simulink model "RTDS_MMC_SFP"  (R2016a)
settings: Solver=FixedStepAuto  StartTime=0.0  StopTime=0.4  RelTol=1e-3
PreLoadFcn:
  | % --- DO NOT REMOVE THIS CODE (2024.3.b1) ---
  |     % create Simulink variants
  |     if not(exist('variant_simulation', 'var'))
  |         variant_simulation = Simulink.Variant('SIMULINK_MODE==0');
  |     end
  |     if not(exist('variant_generation', 'var'))
  |         variant_generation = Simulink.Variant('SIMULINK_MODE==1');
  |     end
  | 
  |     % check SDK version
  |     required_lib_version = 3900.3;
  |     required_lib_ver_str = '2024.3';
  |     lib_path = [getenv('IX_SIMULINK_ACG_BB_3') '\simulink\blocks\BoomBox.slx'];
  |     if exist(lib_path, 'file')
  |         lib_version = str2double(Simulink.MDLInfo(lib_path).ModelVersion); % fullpath to avoid getting shadowing files
  |         if lib_version < required_lib_version || isnan(lib_version)
  |             error(['The model ''' bdroot ''' has been saved with a more recent version of ACG SDK (' required_lib_ver_str ') and might not work as expected. <a href="matlab:private_end_string = ''--- PLACE YOUR CODE BELOW THIS LINE ---'';private_fcn = get_param(bdroot, ''PreLoadFcn'');private_end_index = strfind(private_fcn, private_end_string);set_param(bdroot, ''PreLoadFcn'', strtrim(private_fcn(private_end_index(end)+length(private_end_string):end)));private_fcn = get_param(bdroot, ''PostLoadFcn'');private_end_index = strfind(private_fcn, private_end_string);set_param(bdroot, ''PostLoadFcn'', strtrim(private_fcn(private_end_index(end)+length(private_end_string):end)));private_fcn = get_param(bdroot, ''InitFcn'');private_end_index = strfind(private_fcn, private_end_string);set_param(bdroot, ''InitFcn'', strtrim(private_fcn(private_end_index(end)+length(private_end_string):end)));clear private_end_string private_fcn private_end_index;open(bdroot);">Click here</a> to continue anyway, or download the latest version of the SDK at <a href="www.imperix.com/downloads">www.imperix.ch/downloads</a>.']);
  |         end
  |     elseif exist(getenv('IX_SIMULINK_ACG_BB_3'), 'dir')
  |         error(['Library file for imperix ACG SDK not found in path ''' lib_path '''. Please try to re-install ACG SDK (<a href="www.imperix.com/downloads">www.imperix.ch/downloads</a>).']);
  |     else
  |         error('ACG SDK is not installed on this computer and the model will not work as expected. Please download ACG SDK at <a href="www.imperix.com/downloads">www.imperix.ch/downloads</a>, install it, and reopen the model.');
  |     end
  |     clear required_lib_version required_lib_ver_str lib_path lib_version;
  | 
  |     ix_acg_path = getenv('IX_SIMULINK_ACG_BB_3');
  |     addpath(fullfile(ix_acg_path, 'simulink\target'));
  |     addpath(fullfile(ix_acg_path, 'simulink\blocks'));
  |     addpath(fullfile(ix_acg_path, 'simulink\functions'));
  |     sl_refresh_customizations;
  |     clear ix_acg_path;
  | 
  |     % The SIMULINK_MODE variable is created in the base
  |     % workspace in the PostLoadFcn from the block whose id is kb0101
  |     % All opened models share a common variant configuration.
  | 
  |     Model_PreLoadFcn(bdroot);
  | % --- PLACE YOUR CODE BELOW THIS LINE ---
PostLoadFcn:
  | % --- DO NOT REMOVE THIS CODE (2024.3.b1) ---
  |     % change the execution mode of simulink depending on the radio button:
  |     if(strcmp('Automated Code Generation',get_param(Find_imperix_blocks(bdroot,'Configuration'),'SLMODE')))
  |         assignin('base', 'SIMULINK_MODE', 1);
  |     else
  |         assignin('base', 'SIMULINK_MODE', 0);
  |     end
  | 
  |     Model_PostLoadFcn(bdroot);
  | % --- PLACE YOUR CODE BELOW THIS LINE ---
InitFcn:
  | % --- DO NOT REMOVE THIS CODE (2024.3.b1) ---
  |     % check SDK version
  |     required_lib_version = 3900.3;
  |     required_lib_ver_str = '2024.3';
  |     lib_path = [getenv('IX_SIMULINK_ACG_BB_3') '\simulink\blocks\BoomBox.slx'];
  |     if exist(lib_path, 'file')
  |         lib_version = str2double(Simulink.MDLInfo(lib_path).ModelVersion); % fullpath to avoid getting shadowing files
  |         if lib_version < required_lib_version || isnan(lib_version)
  |             error(['The model ''' bdroot ''' has been saved with a more recent version of ACG SDK (' required_lib_ver_str ') and might not work as expected. <a href="matlab:private_end_string = ''--- PLACE YOUR CODE BELOW THIS LINE ---'';private_fcn = get_param(bdroot, ''PreLoadFcn'');private_end_index = strfind(private_fcn, private_end_string);set_param(bdroot, ''PreLoadFcn'', strtrim(private_fcn(private_end_index(end)+length(private_end_string):end)));private_fcn = get_param(bdroot, ''PostLoadFcn'');private_end_index = strfind(private_fcn, private_end_string);set_param(bdroot, ''PostLoadFcn'', strtrim(private_fcn(private_end_index(end)+length(private_end_string):end)));private_fcn = get_param(bdroot, ''InitFcn'');private_end_index = strfind(private_fcn, private_end_string);set_param(bdroot, ''InitFcn'', strtrim(private_fcn(private_end_index(end)+length(private_end_string):end)));clear private_end_string private_fcn private_end_index;open(bdroot);">Click here</a> to continue anyway, or download the latest version of the SDK at <a href="www.imperix.com/downloads">www.imperix.ch/downloads</a>.']);
  |         end
  |     elseif exist(getenv('IX_SIMULINK_ACG_BB_3'), 'dir')
  |         error(['Library file for imperix ACG SDK not found in path ''' lib_path '''. Please try to re-install ACG SDK (<a href="www.imperix.com/downloads">www.imperix.ch/downloads</a>).']);
  |     else
  |         error('ACG SDK is not installed on this computer and the model will not work as expected. Please download ACG SDK at <a href="www.imperix.com/downloads">www.imperix.ch/downloads</a>, install it, and reopen the model.');
  |     end
  |     clear required_lib_version required_lib_ver_str lib_path lib_version;
  | 
  |     Model_InitFcn(bdroot);
  | % --- PLACE YOUR CODE BELOW THIS LINE ---
model workspace (MAT data in the model file):
  CTRLPERIOD = 0.0002
  TSAMPLE = 2e-06
  global_CLK_number = 0
  global_INT_number = 1
  global_SVM_instance_id = 0
  global_can_baud_rate = '1000000'
  global_comp_time = 0.2
  global_cycle_delay = 8e-05
  global_ip_addresses : cell (value not decoded)
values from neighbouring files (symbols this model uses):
  Ki_Vleg = 1/Ti    (= 2.95256991686)    [RTDS_MMC_SFP_init.m]
  Kp_Vleg = Tn/Ti    (= 0.14880952381)    [RTDS_MMC_SFP_init.m]
  N = 4    [RTDS_MMC_SFP_init.m]
  scale_factor = 0.5^16    (= 1.52587890625e-05)    [RTDS_MMC_SFP_init.m]
  Tsw = 1/fsw    (= 0.0008)    [RTDS_MMC_SFP_init.m]
  Vsm_max = 250    [RTDS_MMC_SFP_init.m]
undefined symbols (not defined in the file or in its folder): B, Board, Box, channel, DT, lane, Micro, ns, PRO, RCP, TPI, Vf
libraries: BoomBox x183, simulink x55
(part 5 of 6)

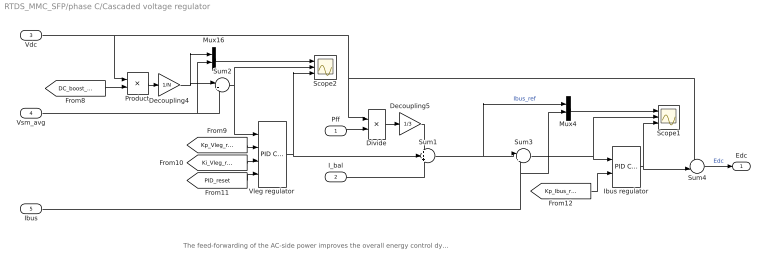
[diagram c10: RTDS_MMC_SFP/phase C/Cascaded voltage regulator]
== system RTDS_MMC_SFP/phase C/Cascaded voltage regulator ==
  note: The feed-forwarding of the AC-side power improves the overall energy control dynamics.
  Pff : Inport
  I_bal : Inport  Port=2
  Vdc : Inport  Port=3
  Vsm_avg : Inport  Port=4
  Ibus : Inport  Port=5
  Decoupling4 : Gain  Gain=1/N
  Decoupling5 : Gain  Gain=1/3
  Divide : Product  Inputs=/*
  Ibus regulator : simulink/Continuous/PID Controller  Controller=P  TimeDomain=Discrete-time  SampleTime=-1  IntegratorMethod=Forward Euler  FilterMethod=Forward Euler  Form=Parallel  UseFilter=on  ControllerParametersSource=external  P=8  I=0.5  D=0  N=100  InitialConditionSource=internal  InitialConditionForIntegrator=0  InitialConditionForFilter=0  ExternalReset=none  LimitOutput=off  UpperSaturationLimit=inf  LowerSaturationLimit=-inf  LinearizeAsGain=off  AntiWindupMode=none  Kb=1  TrackingMode=off  Kt=1  PParamMin=[]  PParamMax=[]  IParamMin=[]  IParamMax=[]  DParamMin=[]  DParamMax=[]  NParamMin=[]  NParamMax=[]  KbParamMin=[]  KbParamMax=[]  KtParamMin=[]  KtParamMax=[]  POutMin=[]  POutMax=[]  IOutMin=[]  IOutMax=[]  DOutMin=[]  DOutMax=[]  NOutMin=[]  NOutMax=[]  KbOutMin=[]  KbOutMax=[]  KtOutMin=[]  KtOutMax=[]  IntegratorOutMin=[]  IntegratorOutMax=[]  FilterOutMin=[]  FilterOutMax=[]  SumOutMin=[]  SumOutMax=[]  SumI1OutMin=[]  SumI1OutMax=[]  SumI2OutMin=[]  SumI2OutMax=[]  SumI3OutMin=[]  SumI3OutMax=[]  SumDOutMin=[]  SumDOutMax=[]  SaturationOutMin=[]  SaturationOutMax=[]  IntegratorContinuousStateAttributes=''  IntegratorStateMustResolveToSignalObject=off  IntegratorRTWStateStorageClass=Auto  FilterContinuousStateAttributes=''  FilterStateMustResolveToSignalObject=off  FilterRTWStateStorageClass=Auto  DifferentiatorICPrevScaledInput=0  DifferentiatorOutMin=[]  DifferentiatorOutMax=[]
  Mux16 : Mux  Inputs=2
  Mux4 : Mux  Inputs=2
  Product : Product
  Scope1 : Scope  NumInputPorts=3
  Scope2 : Scope  NumInputPorts=3
  Sum1 : Sum  Inputs=+++
  Sum2 : Sum  Inputs=|+-
  Sum3 : Sum  Inputs=|+-
  Sum4 : Sum  Inputs=+-|
  Vleg regulator : simulink/Continuous/PID Controller  Controller=PI  TimeDomain=Discrete-time  SampleTime=-1  IntegratorMethod=Forward Euler  FilterMethod=Forward Euler  Form=Parallel  UseFilter=on  ControllerParametersSource=external  P=8  I=0.5  D=0  N=100  InitialConditionSource=internal  InitialConditionForIntegrator=0  InitialConditionForFilter=0  ExternalReset=level  LimitOutput=on  UpperSaturationLimit=10  LowerSaturationLimit=-10  LinearizeAsGain=off  AntiWindupMode=back-calculation  Kb=Ki_Vleg/Kp_Vleg  TrackingMode=off  Kt=1  PParamMin=[]  PParamMax=[]  IParamMin=[]  IParamMax=[]  DParamMin=[]  DParamMax=[]  NParamMin=[]  NParamMax=[]  KbParamMin=[]  KbParamMax=[]  KtParamMin=[]  KtParamMax=[]  POutMin=[]  POutMax=[]  IOutMin=[]  IOutMax=[]  DOutMin=[]  DOutMax=[]  NOutMin=[]  NOutMax=[]  KbOutMin=[]  KbOutMax=[]  KtOutMin=[]  KtOutMax=[]  IntegratorOutMin=[]  IntegratorOutMax=[]  FilterOutMin=[]  FilterOutMax=[]  SumOutMin=[]  SumOutMax=[]  SumI1OutMin=[]  SumI1OutMax=[]  SumI2OutMin=[]  SumI2OutMax=[]  SumI3OutMin=[]  SumI3OutMax=[]  SumDOutMin=[]  SumDOutMax=[]  SaturationOutMin=[]  SaturationOutMax=[]  IntegratorContinuousStateAttributes=''  IntegratorStateMustResolveToSignalObject=off  IntegratorRTWStateStorageClass=Auto  FilterContinuousStateAttributes=''  FilterStateMustResolveToSignalObject=off  FilterRTWStateStorageClass=Auto  DifferentiatorICPrevScaledInput=0  DifferentiatorOutMin=[]  DifferentiatorOutMax=[]
  Edc : Outport
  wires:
  Vdc/1 -> Sum4/1, Divide/1, Product/1
  [PID_reset] -> Vleg regulator/4
  Ibus regulator/1 -> Scope1/3, Sum4/2
  I_bal/1 -> Sum1/3
  [Kp_Ibus_reg] -> Ibus regulator/2
  Pff/1 -> Divide/2
  Vleg regulator/1 -> Sum1/2, Scope2/3
  [Ki_Vleg_reg] -> Vleg regulator/3
  Decoupling5/1 -> Sum1/1
  Mux4/1 -> Scope1/1
  Sum3/1 -> Scope1/2, Ibus regulator/1
  Sum2/1 -> Vleg regulator/1, Scope2/2
  Product/1 -> Decoupling4/1
  Decoupling4/1 -> Mux16/1, Sum2/1
  Sum1/1 -> Sum3/1, Mux4/1  "Ibus_ref"
  Sum4/1 -> Edc/1  "Edc"
  [DC_boost_ratio] -> Product/2
  Vsm_avg/1 -> Mux16/2, Sum2/2
  Divide/1 -> Decoupling5/1
  Mux16/1 -> Scope2/1
  Ibus/1 -> Sum3/2, Mux4/2
  [Kp_Vleg_reg] -> Vleg regulator/2

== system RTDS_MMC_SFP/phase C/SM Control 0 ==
  Vsm : Inport
  sign : Inport  Port=2
  Vsm_avg : Inport  Port=3
  Eac : Inport  Port=4
  Edc : Inport  Port=5
  Decoupling1 : Gain  Gain=1/(2*N)
  Decoupling2 : Gain  Gain=1/(N)
  Divide6 : Product  Inputs=/*
  Divide7 : Product  Inputs=**
  Saturation : Saturate  UpperLimit=0.95  LowerLimit=0.05
  Sum1 : Sum  Inputs=|++
  Sum2 : Sum  Inputs=-+|
  Sum3 : Sum  Inputs=|++
  Vsm regulator : simulink/Continuous/PID Controller  Controller=P  TimeDomain=Discrete-time  SampleTime=-1  IntegratorMethod=Forward Euler  FilterMethod=Forward Euler  Form=Parallel  UseFilter=on  ControllerParametersSource=external  P=8  I=0.5  D=0  N=100  InitialConditionSource=internal  InitialConditionForIntegrator=0  InitialConditionForFilter=0  ExternalReset=none  LimitOutput=off  UpperSaturationLimit=inf  LowerSaturationLimit=-inf  LinearizeAsGain=off  AntiWindupMode=none  Kb=1  TrackingMode=off  Kt=1  PParamMin=[]  PParamMax=[]  IParamMin=[]  IParamMax=[]  DParamMin=[]  DParamMax=[]  NParamMin=[]  NParamMax=[]  KbParamMin=[]  KbParamMax=[]  KtParamMin=[]  KtParamMax=[]  POutMin=[]  POutMax=[]  IOutMin=[]  IOutMax=[]  DOutMin=[]  DOutMax=[]  NOutMin=[]  NOutMax=[]  KbOutMin=[]  KbOutMax=[]  KtOutMin=[]  KtOutMax=[]  IntegratorOutMin=[]  IntegratorOutMax=[]  FilterOutMin=[]  FilterOutMax=[]  SumOutMin=[]  SumOutMax=[]  SumI1OutMin=[]  SumI1OutMax=[]  SumI2OutMin=[]  SumI2OutMax=[]  SumI3OutMin=[]  SumI3OutMax=[]  SumDOutMin=[]  SumDOutMax=[]  SaturationOutMin=[]  SaturationOutMax=[]  IntegratorContinuousStateAttributes=''  IntegratorStateMustResolveToSignalObject=off  IntegratorRTWStateStorageClass=Auto  FilterContinuousStateAttributes=''  FilterStateMustResolveToSignalObject=off  FilterRTWStateStorageClass=Auto  DifferentiatorICPrevScaledInput=0  DifferentiatorOutMin=[]  DifferentiatorOutMax=[]
  dead time compensation : Subsystem
  m : Outport
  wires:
  [Kp_Vsm_reg] -> Vsm regulator/2
  Sum2/1 -> Vsm regulator/1
  sign/1 -> dead time compensation/1(sign), Divide7/1
  Vsm regulator/1 -> Divide7/2
  Vsm/1 -> dead time compensation/2(Vdc), Divide6/1, Sum2/1
  Vsm_avg/1 -> Sum2/2
  Sum3/1 -> Divide6/2
  Saturation/1 -> m/1
  Divide6/1 -> dead time compensation/3(m)  "m"
  dead time compensation/1(m') -> Saturation/1
  Divide7/1 -> Sum1/1
  Sum1/1 -> Sum3/1
  Eac/1 -> Decoupling2/1
  Decoupling2/1 -> Sum1/2
  Edc/1 -> Decoupling1/1
  Decoupling1/1 -> Sum3/2

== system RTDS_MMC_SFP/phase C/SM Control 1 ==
  Vsm : Inport
  sign : Inport  Port=2
  Vsm_avg : Inport  Port=3
  Eac : Inport  Port=4
  Edc : Inport  Port=5
  Decoupling1 : Gain  Gain=1/(2*N)
  Decoupling2 : Gain  Gain=1/(N)
  Divide6 : Product  Inputs=/*
  Divide7 : Product  Inputs=**
  Saturation : Saturate  UpperLimit=0.95  LowerLimit=0.05
  Sum1 : Sum  Inputs=|++
  Sum2 : Sum  Inputs=-+|
  Sum3 : Sum  Inputs=|++
  Vsm regulator : simulink/Continuous/PID Controller  Controller=P  TimeDomain=Discrete-time  SampleTime=-1  IntegratorMethod=Forward Euler  FilterMethod=Forward Euler  Form=Parallel  UseFilter=on  ControllerParametersSource=external  P=8  I=0.5  D=0  N=100  InitialConditionSource=internal  InitialConditionForIntegrator=0  InitialConditionForFilter=0  ExternalReset=none  LimitOutput=off  UpperSaturationLimit=inf  LowerSaturationLimit=-inf  LinearizeAsGain=off  AntiWindupMode=none  Kb=1  TrackingMode=off  Kt=1  PParamMin=[]  PParamMax=[]  IParamMin=[]  IParamMax=[]  DParamMin=[]  DParamMax=[]  NParamMin=[]  NParamMax=[]  KbParamMin=[]  KbParamMax=[]  KtParamMin=[]  KtParamMax=[]  POutMin=[]  POutMax=[]  IOutMin=[]  IOutMax=[]  DOutMin=[]  DOutMax=[]  NOutMin=[]  NOutMax=[]  KbOutMin=[]  KbOutMax=[]  KtOutMin=[]  KtOutMax=[]  IntegratorOutMin=[]  IntegratorOutMax=[]  FilterOutMin=[]  FilterOutMax=[]  SumOutMin=[]  SumOutMax=[]  SumI1OutMin=[]  SumI1OutMax=[]  SumI2OutMin=[]  SumI2OutMax=[]  SumI3OutMin=[]  SumI3OutMax=[]  SumDOutMin=[]  SumDOutMax=[]  SaturationOutMin=[]  SaturationOutMax=[]  IntegratorContinuousStateAttributes=''  IntegratorStateMustResolveToSignalObject=off  IntegratorRTWStateStorageClass=Auto  FilterContinuousStateAttributes=''  FilterStateMustResolveToSignalObject=off  FilterRTWStateStorageClass=Auto  DifferentiatorICPrevScaledInput=0  DifferentiatorOutMin=[]  DifferentiatorOutMax=[]
  dead time compensation : Subsystem
  m : Outport
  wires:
  Decoupling1/1 -> Sum3/2
  Edc/1 -> Decoupling1/1
  Decoupling2/1 -> Sum1/2
  Eac/1 -> Decoupling2/1
  Sum1/1 -> Sum3/1
  Divide7/1 -> Sum1/1
  dead time compensation/1(m') -> Saturation/1
  Divide6/1 -> dead time compensation/3(m)  "m"
  Saturation/1 -> m/1
  Sum3/1 -> Divide6/2
  Vsm_avg/1 -> Sum2/2
  Vsm/1 -> Sum2/1, Divide6/1, dead time compensation/2(Vdc)
  Vsm regulator/1 -> Divide7/2
  sign/1 -> Divide7/1, dead time compensation/1(sign)
  Sum2/1 -> Vsm regulator/1
  [Kp_Vsm_reg] -> Vsm regulator/2

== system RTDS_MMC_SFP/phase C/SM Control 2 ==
  Vsm : Inport
  sign : Inport  Port=2
  Vsm_avg : Inport  Port=3
  Eac : Inport  Port=4
  Edc : Inport  Port=5
  Decoupling1 : Gain  Gain=1/(2*N)
  Decoupling2 : Gain  Gain=1/(N)
  Divide6 : Product  Inputs=/*
  Divide7 : Product  Inputs=**
  Saturation : Saturate  UpperLimit=0.95  LowerLimit=0.05
  Sum1 : Sum  Inputs=|++
  Sum2 : Sum  Inputs=-+|
  Sum3 : Sum  Inputs=|++
  Vsm regulator : simulink/Continuous/PID Controller  Controller=P  TimeDomain=Discrete-time  SampleTime=-1  IntegratorMethod=Forward Euler  FilterMethod=Forward Euler  Form=Parallel  UseFilter=on  ControllerParametersSource=external  P=8  I=0.5  D=0  N=100  InitialConditionSource=internal  InitialConditionForIntegrator=0  InitialConditionForFilter=0  ExternalReset=none  LimitOutput=off  UpperSaturationLimit=inf  LowerSaturationLimit=-inf  LinearizeAsGain=off  AntiWindupMode=none  Kb=1  TrackingMode=off  Kt=1  PParamMin=[]  PParamMax=[]  IParamMin=[]  IParamMax=[]  DParamMin=[]  DParamMax=[]  NParamMin=[]  NParamMax=[]  KbParamMin=[]  KbParamMax=[]  KtParamMin=[]  KtParamMax=[]  POutMin=[]  POutMax=[]  IOutMin=[]  IOutMax=[]  DOutMin=[]  DOutMax=[]  NOutMin=[]  NOutMax=[]  KbOutMin=[]  KbOutMax=[]  KtOutMin=[]  KtOutMax=[]  IntegratorOutMin=[]  IntegratorOutMax=[]  FilterOutMin=[]  FilterOutMax=[]  SumOutMin=[]  SumOutMax=[]  SumI1OutMin=[]  SumI1OutMax=[]  SumI2OutMin=[]  SumI2OutMax=[]  SumI3OutMin=[]  SumI3OutMax=[]  SumDOutMin=[]  SumDOutMax=[]  SaturationOutMin=[]  SaturationOutMax=[]  IntegratorContinuousStateAttributes=''  IntegratorStateMustResolveToSignalObject=off  IntegratorRTWStateStorageClass=Auto  FilterContinuousStateAttributes=''  FilterStateMustResolveToSignalObject=off  FilterRTWStateStorageClass=Auto  DifferentiatorICPrevScaledInput=0  DifferentiatorOutMin=[]  DifferentiatorOutMax=[]
  dead time compensation : Subsystem
  m : Outport
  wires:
  [Kp_Vsm_reg] -> Vsm regulator/2
  Sum2/1 -> Vsm regulator/1
  sign/1 -> dead time compensation/1(sign), Divide7/1
  Vsm regulator/1 -> Divide7/2
  Vsm/1 -> dead time compensation/2(Vdc), Divide6/1, Sum2/1
  Vsm_avg/1 -> Sum2/2
  Sum3/1 -> Divide6/2
  Saturation/1 -> m/1
  Divide6/1 -> dead time compensation/3(m)  "m"
  dead time compensation/1(m') -> Saturation/1
  Divide7/1 -> Sum1/1
  Sum1/1 -> Sum3/1
  Eac/1 -> Decoupling2/1
  Decoupling2/1 -> Sum1/2
  Edc/1 -> Decoupling1/1
  Decoupling1/1 -> Sum3/2

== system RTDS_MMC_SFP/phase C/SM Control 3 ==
  Vsm : Inport
  sign : Inport  Port=2
  Vsm_avg : Inport  Port=3
  Eac : Inport  Port=4
  Edc : Inport  Port=5
  Decoupling1 : Gain  Gain=1/(2*N)
  Decoupling2 : Gain  Gain=1/(N)
  Divide6 : Product  Inputs=/*
  Divide7 : Product  Inputs=**
  Saturation : Saturate  UpperLimit=0.95  LowerLimit=0.05
  Sum1 : Sum  Inputs=|++
  Sum2 : Sum  Inputs=-+|
  Sum3 : Sum  Inputs=|++
  Vsm regulator : simulink/Continuous/PID Controller  Controller=P  TimeDomain=Discrete-time  SampleTime=-1  IntegratorMethod=Forward Euler  FilterMethod=Forward Euler  Form=Parallel  UseFilter=on  ControllerParametersSource=external  P=8  I=0.5  D=0  N=100  InitialConditionSource=internal  InitialConditionForIntegrator=0  InitialConditionForFilter=0  ExternalReset=none  LimitOutput=off  UpperSaturationLimit=inf  LowerSaturationLimit=-inf  LinearizeAsGain=off  AntiWindupMode=none  Kb=1  TrackingMode=off  Kt=1  PParamMin=[]  PParamMax=[]  IParamMin=[]  IParamMax=[]  DParamMin=[]  DParamMax=[]  NParamMin=[]  NParamMax=[]  KbParamMin=[]  KbParamMax=[]  KtParamMin=[]  KtParamMax=[]  POutMin=[]  POutMax=[]  IOutMin=[]  IOutMax=[]  DOutMin=[]  DOutMax=[]  NOutMin=[]  NOutMax=[]  KbOutMin=[]  KbOutMax=[]  KtOutMin=[]  KtOutMax=[]  IntegratorOutMin=[]  IntegratorOutMax=[]  FilterOutMin=[]  FilterOutMax=[]  SumOutMin=[]  SumOutMax=[]  SumI1OutMin=[]  SumI1OutMax=[]  SumI2OutMin=[]  SumI2OutMax=[]  SumI3OutMin=[]  SumI3OutMax=[]  SumDOutMin=[]  SumDOutMax=[]  SaturationOutMin=[]  SaturationOutMax=[]  IntegratorContinuousStateAttributes=''  IntegratorStateMustResolveToSignalObject=off  IntegratorRTWStateStorageClass=Auto  FilterContinuousStateAttributes=''  FilterStateMustResolveToSignalObject=off  FilterRTWStateStorageClass=Auto  DifferentiatorICPrevScaledInput=0  DifferentiatorOutMin=[]  DifferentiatorOutMax=[]
  dead time compensation : Subsystem
  m : Outport
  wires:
  Decoupling1/1 -> Sum3/2
  Edc/1 -> Decoupling1/1
  Decoupling2/1 -> Sum1/2
  Eac/1 -> Decoupling2/1
  Sum1/1 -> Sum3/1
  Divide7/1 -> Sum1/1
  dead time compensation/1(m') -> Saturation/1
  Divide6/1 -> dead time compensation/3(m)  "m"
  Saturation/1 -> m/1
  Sum3/1 -> Divide6/2
  Vsm_avg/1 -> Sum2/2
  Vsm/1 -> Sum2/1, Divide6/1, dead time compensation/2(Vdc)
  Vsm regulator/1 -> Divide7/2
  sign/1 -> Divide7/1, dead time compensation/1(sign)
  Sum2/1 -> Vsm regulator/1
  [Kp_Vsm_reg] -> Vsm regulator/2

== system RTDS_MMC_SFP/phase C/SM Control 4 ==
  Vsm : Inport
  sign : Inport  Port=2
  Vsm_avg : Inport  Port=3
  Eac : Inport  Port=4
  Edc : Inport  Port=5
  Decoupling1 : Gain  Gain=1/(2*N)
  Decoupling2 : Gain  Gain=1/(N)
  Divide6 : Product  Inputs=/*
  Divide7 : Product  Inputs=**
  Saturation : Saturate  UpperLimit=0.95  LowerLimit=0.05
  Sum1 : Sum  Inputs=|++
  Sum2 : Sum  Inputs=-+|
  Sum3 : Sum  Inputs=|++
  Vsm regulator : simulink/Continuous/PID Controller  Controller=P  TimeDomain=Discrete-time  SampleTime=-1  IntegratorMethod=Forward Euler  FilterMethod=Forward Euler  Form=Parallel  UseFilter=on  ControllerParametersSource=external  P=8  I=0.5  D=0  N=100  InitialConditionSource=internal  InitialConditionForIntegrator=0  InitialConditionForFilter=0  ExternalReset=none  LimitOutput=off  UpperSaturationLimit=inf  LowerSaturationLimit=-inf  LinearizeAsGain=off  AntiWindupMode=none  Kb=1  TrackingMode=off  Kt=1  PParamMin=[]  PParamMax=[]  IParamMin=[]  IParamMax=[]  DParamMin=[]  DParamMax=[]  NParamMin=[]  NParamMax=[]  KbParamMin=[]  KbParamMax=[]  KtParamMin=[]  KtParamMax=[]  POutMin=[]  POutMax=[]  IOutMin=[]  IOutMax=[]  DOutMin=[]  DOutMax=[]  NOutMin=[]  NOutMax=[]  KbOutMin=[]  KbOutMax=[]  KtOutMin=[]  KtOutMax=[]  IntegratorOutMin=[]  IntegratorOutMax=[]  FilterOutMin=[]  FilterOutMax=[]  SumOutMin=[]  SumOutMax=[]  SumI1OutMin=[]  SumI1OutMax=[]  SumI2OutMin=[]  SumI2OutMax=[]  SumI3OutMin=[]  SumI3OutMax=[]  SumDOutMin=[]  SumDOutMax=[]  SaturationOutMin=[]  SaturationOutMax=[]  IntegratorContinuousStateAttributes=''  IntegratorStateMustResolveToSignalObject=off  IntegratorRTWStateStorageClass=Auto  FilterContinuousStateAttributes=''  FilterStateMustResolveToSignalObject=off  FilterRTWStateStorageClass=Auto  DifferentiatorICPrevScaledInput=0  DifferentiatorOutMin=[]  DifferentiatorOutMax=[]
  dead time compensation : Subsystem
  m : Outport
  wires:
  Decoupling1/1 -> Sum3/2
  Edc/1 -> Decoupling1/1
  Decoupling2/1 -> Sum1/2
  Eac/1 -> Decoupling2/1
  Sum1/1 -> Sum3/1
  Divide7/1 -> Sum1/1
  dead time compensation/1(m') -> Saturation/1
  Divide6/1 -> dead time compensation/3(m)  "m"
  Saturation/1 -> m/1
  Sum3/1 -> Divide6/2
  Vsm_avg/1 -> Sum2/2
  Vsm/1 -> Sum2/1, Divide6/1, dead time compensation/2(Vdc)
  Vsm regulator/1 -> Divide7/2
  sign/1 -> Divide7/1, dead time compensation/1(sign)
  Sum2/1 -> Vsm regulator/1
  [Kp_Vsm_reg] -> Vsm regulator/2

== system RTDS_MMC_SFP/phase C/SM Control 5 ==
  Vsm : Inport
  sign : Inport  Port=2
  Vsm_avg : Inport  Port=3
  Eac : Inport  Port=4
  Edc : Inport  Port=5
  Decoupling1 : Gain  Gain=1/(2*N)
  Decoupling2 : Gain  Gain=1/(N)
  Divide6 : Product  Inputs=/*
  Divide7 : Product  Inputs=**
  Saturation : Saturate  UpperLimit=0.95  LowerLimit=0.05
  Sum1 : Sum  Inputs=|++
  Sum2 : Sum  Inputs=-+|
  Sum3 : Sum  Inputs=|++
  Vsm regulator : simulink/Continuous/PID Controller  Controller=P  TimeDomain=Discrete-time  SampleTime=-1  IntegratorMethod=Forward Euler  FilterMethod=Forward Euler  Form=Parallel  UseFilter=on  ControllerParametersSource=external  P=8  I=0.5  D=0  N=100  InitialConditionSource=internal  InitialConditionForIntegrator=0  InitialConditionForFilter=0  ExternalReset=none  LimitOutput=off  UpperSaturationLimit=inf  LowerSaturationLimit=-inf  LinearizeAsGain=off  AntiWindupMode=none  Kb=1  TrackingMode=off  Kt=1  PParamMin=[]  PParamMax=[]  IParamMin=[]  IParamMax=[]  DParamMin=[]  DParamMax=[]  NParamMin=[]  NParamMax=[]  KbParamMin=[]  KbParamMax=[]  KtParamMin=[]  KtParamMax=[]  POutMin=[]  POutMax=[]  IOutMin=[]  IOutMax=[]  DOutMin=[]  DOutMax=[]  NOutMin=[]  NOutMax=[]  KbOutMin=[]  KbOutMax=[]  KtOutMin=[]  KtOutMax=[]  IntegratorOutMin=[]  IntegratorOutMax=[]  FilterOutMin=[]  FilterOutMax=[]  SumOutMin=[]  SumOutMax=[]  SumI1OutMin=[]  SumI1OutMax=[]  SumI2OutMin=[]  SumI2OutMax=[]  SumI3OutMin=[]  SumI3OutMax=[]  SumDOutMin=[]  SumDOutMax=[]  SaturationOutMin=[]  SaturationOutMax=[]  IntegratorContinuousStateAttributes=''  IntegratorStateMustResolveToSignalObject=off  IntegratorRTWStateStorageClass=Auto  FilterContinuousStateAttributes=''  FilterStateMustResolveToSignalObject=off  FilterRTWStateStorageClass=Auto  DifferentiatorICPrevScaledInput=0  DifferentiatorOutMin=[]  DifferentiatorOutMax=[]
  dead time compensation : Subsystem
  m : Outport
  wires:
  [Kp_Vsm_reg] -> Vsm regulator/2
  Sum2/1 -> Vsm regulator/1
  sign/1 -> dead time compensation/1(sign), Divide7/1
  Vsm regulator/1 -> Divide7/2
  Vsm/1 -> dead time compensation/2(Vdc), Divide6/1, Sum2/1
  Vsm_avg/1 -> Sum2/2
  Sum3/1 -> Divide6/2
  Saturation/1 -> m/1
  Divide6/1 -> dead time compensation/3(m)  "m"
  dead time compensation/1(m') -> Saturation/1
  Divide7/1 -> Sum1/1
  Sum1/1 -> Sum3/1
  Eac/1 -> Decoupling2/1
  Decoupling2/1 -> Sum1/2
  Edc/1 -> Decoupling1/1
  Decoupling1/1 -> Sum3/2

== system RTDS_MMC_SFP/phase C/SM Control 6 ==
  Vsm : Inport
  sign : Inport  Port=2
  Vsm_avg : Inport  Port=3
  Eac : Inport  Port=4
  Edc : Inport  Port=5
  Decoupling1 : Gain  Gain=1/(2*N)
  Decoupling2 : Gain  Gain=1/(N)
  Divide6 : Product  Inputs=/*
  Divide7 : Product  Inputs=**
  Saturation : Saturate  UpperLimit=0.95  LowerLimit=0.05
  Sum1 : Sum  Inputs=|++
  Sum2 : Sum  Inputs=-+|
  Sum3 : Sum  Inputs=|++
  Vsm regulator : simulink/Continuous/PID Controller  Controller=P  TimeDomain=Discrete-time  SampleTime=-1  IntegratorMethod=Forward Euler  FilterMethod=Forward Euler  Form=Parallel  UseFilter=on  ControllerParametersSource=external  P=8  I=0.5  D=0  N=100  InitialConditionSource=internal  InitialConditionForIntegrator=0  InitialConditionForFilter=0  ExternalReset=none  LimitOutput=off  UpperSaturationLimit=inf  LowerSaturationLimit=-inf  LinearizeAsGain=off  AntiWindupMode=none  Kb=1  TrackingMode=off  Kt=1  PParamMin=[]  PParamMax=[]  IParamMin=[]  IParamMax=[]  DParamMin=[]  DParamMax=[]  NParamMin=[]  NParamMax=[]  KbParamMin=[]  KbParamMax=[]  KtParamMin=[]  KtParamMax=[]  POutMin=[]  POutMax=[]  IOutMin=[]  IOutMax=[]  DOutMin=[]  DOutMax=[]  NOutMin=[]  NOutMax=[]  KbOutMin=[]  KbOutMax=[]  KtOutMin=[]  KtOutMax=[]  IntegratorOutMin=[]  IntegratorOutMax=[]  FilterOutMin=[]  FilterOutMax=[]  SumOutMin=[]  SumOutMax=[]  SumI1OutMin=[]  SumI1OutMax=[]  SumI2OutMin=[]  SumI2OutMax=[]  SumI3OutMin=[]  SumI3OutMax=[]  SumDOutMin=[]  SumDOutMax=[]  SaturationOutMin=[]  SaturationOutMax=[]  IntegratorContinuousStateAttributes=''  IntegratorStateMustResolveToSignalObject=off  IntegratorRTWStateStorageClass=Auto  FilterContinuousStateAttributes=''  FilterStateMustResolveToSignalObject=off  FilterRTWStateStorageClass=Auto  DifferentiatorICPrevScaledInput=0  DifferentiatorOutMin=[]  DifferentiatorOutMax=[]
  dead time compensation : Subsystem
  m : Outport
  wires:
  Decoupling1/1 -> Sum3/2
  Edc/1 -> Decoupling1/1
  Decoupling2/1 -> Sum1/2
  Eac/1 -> Decoupling2/1
  Sum1/1 -> Sum3/1
  Divide7/1 -> Sum1/1
  dead time compensation/1(m') -> Saturation/1
  Divide6/1 -> dead time compensation/3(m)  "m"
  Saturation/1 -> m/1
  Sum3/1 -> Divide6/2
  Vsm_avg/1 -> Sum2/2
  Vsm/1 -> Sum2/1, Divide6/1, dead time compensation/2(Vdc)
  Vsm regulator/1 -> Divide7/2
  sign/1 -> Divide7/1, dead time compensation/1(sign)
  Sum2/1 -> Vsm regulator/1
  [Kp_Vsm_reg] -> Vsm regulator/2

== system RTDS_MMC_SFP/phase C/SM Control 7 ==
  Vsm : Inport
  sign : Inport  Port=2
  Vsm_avg : Inport  Port=3
  Eac : Inport  Port=4
  Edc : Inport  Port=5
  Decoupling1 : Gain  Gain=1/(2*N)
  Decoupling2 : Gain  Gain=1/(N)
  Divide6 : Product  Inputs=/*
  Divide7 : Product  Inputs=**
  Saturation : Saturate  UpperLimit=0.95  LowerLimit=0.05
  Sum1 : Sum  Inputs=|++
  Sum2 : Sum  Inputs=-+|
  Sum3 : Sum  Inputs=|++
  Vsm regulator : simulink/Continuous/PID Controller  Controller=P  TimeDomain=Discrete-time  SampleTime=-1  IntegratorMethod=Forward Euler  FilterMethod=Forward Euler  Form=Parallel  UseFilter=on  ControllerParametersSource=external  P=8  I=0.5  D=0  N=100  InitialConditionSource=internal  InitialConditionForIntegrator=0  InitialConditionForFilter=0  ExternalReset=none  LimitOutput=off  UpperSaturationLimit=inf  LowerSaturationLimit=-inf  LinearizeAsGain=off  AntiWindupMode=none  Kb=1  TrackingMode=off  Kt=1  PParamMin=[]  PParamMax=[]  IParamMin=[]  IParamMax=[]  DParamMin=[]  DParamMax=[]  NParamMin=[]  NParamMax=[]  KbParamMin=[]  KbParamMax=[]  KtParamMin=[]  KtParamMax=[]  POutMin=[]  POutMax=[]  IOutMin=[]  IOutMax=[]  DOutMin=[]  DOutMax=[]  NOutMin=[]  NOutMax=[]  KbOutMin=[]  KbOutMax=[]  KtOutMin=[]  KtOutMax=[]  IntegratorOutMin=[]  IntegratorOutMax=[]  FilterOutMin=[]  FilterOutMax=[]  SumOutMin=[]  SumOutMax=[]  SumI1OutMin=[]  SumI1OutMax=[]  SumI2OutMin=[]  SumI2OutMax=[]  SumI3OutMin=[]  SumI3OutMax=[]  SumDOutMin=[]  SumDOutMax=[]  SaturationOutMin=[]  SaturationOutMax=[]  IntegratorContinuousStateAttributes=''  IntegratorStateMustResolveToSignalObject=off  IntegratorRTWStateStorageClass=Auto  FilterContinuousStateAttributes=''  FilterStateMustResolveToSignalObject=off  FilterRTWStateStorageClass=Auto  DifferentiatorICPrevScaledInput=0  DifferentiatorOutMin=[]  DifferentiatorOutMax=[]
  dead time compensation : Subsystem
  m : Outport
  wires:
  [Kp_Vsm_reg] -> Vsm regulator/2
  Sum2/1 -> Vsm regulator/1
  sign/1 -> dead time compensation/1(sign), Divide7/1
  Vsm regulator/1 -> Divide7/2
  Vsm/1 -> dead time compensation/2(Vdc), Divide6/1, Sum2/1
  Vsm_avg/1 -> Sum2/2
  Sum3/1 -> Divide6/2
  Saturation/1 -> m/1
  Divide6/1 -> dead time compensation/3(m)  "m"
  dead time compensation/1(m') -> Saturation/1
  Divide7/1 -> Sum1/1
  Sum1/1 -> Sum3/1
  Eac/1 -> Decoupling2/1
  Decoupling2/1 -> Sum1/2
  Edc/1 -> Decoupling1/1
  Decoupling1/1 -> Sum3/2

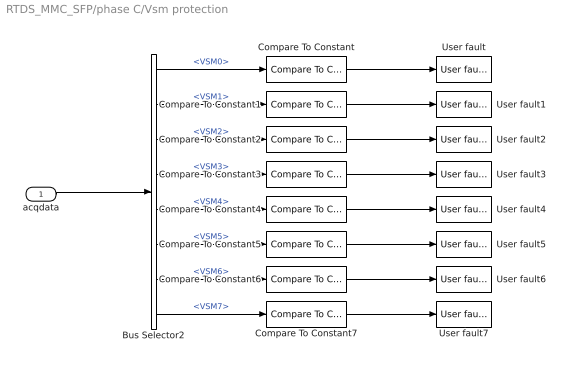
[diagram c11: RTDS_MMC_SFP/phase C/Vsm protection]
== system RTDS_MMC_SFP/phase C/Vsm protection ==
  acqdata : Inport
  Bus Selector2 : BusSelector  OutputSignals=A.Vsm.Vsm_up.VSM0,A.Vsm.Vsm_up.VSM1,A.Vsm.Vsm_up.VSM2,A.Vsm.Vsm_up.VSM3,A.Vsm.Vsm_low.VSM4,A.Vsm.Vsm_low.VSM5,A.Vsm.Vsm_low.VSM6,A.Vsm.Vsm_low.VSM7
  Compare To Constant{,1..7} (8 alike) : simulink/Logic and Bit Operations/Compare To Constant  relop=>  const=Vsm_max  OutDataTypeStr=boolean
  User fault : BoomBox/User fault  MESSAGE=Overvoltage Vsm on module A0  EVALUATE=Literal  KBID=kb0506
  User fault1 : BoomBox/User fault  MESSAGE=Overvoltage Vsm on module A1  EVALUATE=Literal  KBID=kb0506
  User fault2 : BoomBox/User fault  MESSAGE=Overvoltage Vsm on module A2  EVALUATE=Literal  KBID=kb0506
  User fault3 : BoomBox/User fault  MESSAGE=Overvoltage Vsm on module A3  EVALUATE=Literal  KBID=kb0506
  User fault4 : BoomBox/User fault  MESSAGE=Overvoltage Vsm on module A4  EVALUATE=Literal  KBID=kb0506
  User fault5 : BoomBox/User fault  MESSAGE=Overvoltage Vsm on module A5  EVALUATE=Literal  KBID=kb0506
  User fault6 : BoomBox/User fault  MESSAGE=Overvoltage Vsm on module A6  EVALUATE=Literal  KBID=kb0506
  User fault7 : BoomBox/User fault  MESSAGE=Overvoltage Vsm on module A7  EVALUATE=Literal  KBID=kb0506
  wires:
  Bus Selector2/5 -> Compare To Constant4/1  "<VSM4>"
  Bus Selector2/2 -> Compare To Constant1/1  "<VSM1>"
  Bus Selector2/3 -> Compare To Constant2/1  "<VSM2>"
  Bus Selector2/4 -> Compare To Constant3/1  "<VSM3>"
  Bus Selector2/8 -> Compare To Constant7/1  "<VSM7>"
  Bus Selector2/7 -> Compare To Constant6/1  "<VSM6>"
  Bus Selector2/6 -> Compare To Constant5/1  "<VSM5>"
  Bus Selector2/1 -> Compare To Constant/1  "<VSM0>"
  acqdata/1 -> Bus Selector2/1
  Compare To Constant/1 -> User fault/1
  Compare To Constant1/1 -> User fault1/1
  Compare To Constant2/1 -> User fault2/1
  Compare To Constant3/1 -> User fault3/1
  Compare To Constant4/1 -> User fault4/1
  Compare To Constant5/1 -> User fault5/1
  Compare To Constant6/1 -> User fault6/1
  Compare To Constant7/1 -> User fault7/1

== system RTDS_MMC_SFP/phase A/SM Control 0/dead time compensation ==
  sign : Inport
  Vdc : Inport  Port=2
  m : Inport  Port=3
  Constant1 : Constant  Value=Vf  OutDataTypeStr=single
  Constant2 : Constant  Value=DT/Tsw  OutDataTypeStr=single
  Gain : Gain  Gain=0.5
  Product : Product
  Product1 : Product
  Product2 : Product
  Product3 : Product  Inputs=/*
  Sum : Sum  Inputs=|++
  Sum1 : Sum  Inputs=|++
  Sum2 : Sum  Inputs=|++
  m' : Outport
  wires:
  m/1 -> Product1/1, Sum/1
  Sum/1 -> m'/1
  Constant1/1 -> Sum1/2, Product1/2
  Sum1/1 -> Product/1
  Constant2/1 -> Product/2
  Product/1 -> Sum2/1
  Product1/1 -> Sum2/2
  Sum2/1 -> Product2/1
  sign/1 -> Product2/2
  Product2/1 -> Gain/1
  Product3/1 -> Sum/2
  Vdc/1 -> Sum1/1, Product3/1
  Gain/1 -> Product3/2

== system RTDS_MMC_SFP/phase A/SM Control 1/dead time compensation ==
  sign : Inport
  Vdc : Inport  Port=2
  m : Inport  Port=3
  Constant1 : Constant  Value=Vf  OutDataTypeStr=single
  Constant2 : Constant  Value=DT/Tsw  OutDataTypeStr=single
  Gain : Gain  Gain=0.5
  Product : Product
  Product1 : Product
  Product2 : Product
  Product3 : Product  Inputs=/*
  Sum : Sum  Inputs=|++
  Sum1 : Sum  Inputs=|++
  Sum2 : Sum  Inputs=|++
  m' : Outport
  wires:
  Gain/1 -> Product3/2
  Vdc/1 -> Product3/1, Sum1/1
  Product3/1 -> Sum/2
  Product2/1 -> Gain/1
  sign/1 -> Product2/2
  Sum2/1 -> Product2/1
  Product1/1 -> Sum2/2
  Product/1 -> Sum2/1
  Constant2/1 -> Product/2
  Sum1/1 -> Product/1
  Constant1/1 -> Product1/2, Sum1/2
  Sum/1 -> m'/1
  m/1 -> Sum/1, Product1/1

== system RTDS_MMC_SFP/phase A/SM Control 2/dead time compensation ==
  sign : Inport
  Vdc : Inport  Port=2
  m : Inport  Port=3
  Constant1 : Constant  Value=Vf  OutDataTypeStr=single
  Constant2 : Constant  Value=DT/Tsw  OutDataTypeStr=single
  Gain : Gain  Gain=0.5
  Product : Product
  Product1 : Product
  Product2 : Product
  Product3 : Product  Inputs=/*
  Sum : Sum  Inputs=|++
  Sum1 : Sum  Inputs=|++
  Sum2 : Sum  Inputs=|++
  m' : Outport
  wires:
  m/1 -> Product1/1, Sum/1
  Sum/1 -> m'/1
  Constant1/1 -> Sum1/2, Product1/2
  Sum1/1 -> Product/1
  Constant2/1 -> Product/2
  Product/1 -> Sum2/1
  Product1/1 -> Sum2/2
  Sum2/1 -> Product2/1
  sign/1 -> Product2/2
  Product2/1 -> Gain/1
  Product3/1 -> Sum/2
  Vdc/1 -> Sum1/1, Product3/1
  Gain/1 -> Product3/2

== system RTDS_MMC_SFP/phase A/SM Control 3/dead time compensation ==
  sign : Inport
  Vdc : Inport  Port=2
  m : Inport  Port=3
  Constant1 : Constant  Value=Vf  OutDataTypeStr=single
  Constant2 : Constant  Value=DT/Tsw  OutDataTypeStr=single
  Gain : Gain  Gain=0.5
  Product : Product
  Product1 : Product
  Product2 : Product
  Product3 : Product  Inputs=/*
  Sum : Sum  Inputs=|++
  Sum1 : Sum  Inputs=|++
  Sum2 : Sum  Inputs=|++
  m' : Outport
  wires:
  Gain/1 -> Product3/2
  Vdc/1 -> Product3/1, Sum1/1
  Product3/1 -> Sum/2
  Product2/1 -> Gain/1
  sign/1 -> Product2/2
  Sum2/1 -> Product2/1
  Product1/1 -> Sum2/2
  Product/1 -> Sum2/1
  Constant2/1 -> Product/2
  Sum1/1 -> Product/1
  Constant1/1 -> Product1/2, Sum1/2
  Sum/1 -> m'/1
  m/1 -> Sum/1, Product1/1

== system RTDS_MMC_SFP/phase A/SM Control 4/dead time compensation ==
  sign : Inport
  Vdc : Inport  Port=2
  m : Inport  Port=3
  Constant1 : Constant  Value=Vf  OutDataTypeStr=single
  Constant2 : Constant  Value=DT/Tsw  OutDataTypeStr=single
  Gain : Gain  Gain=0.5
  Product : Product
  Product1 : Product
  Product2 : Product
  Product3 : Product  Inputs=/*
  Sum : Sum  Inputs=|++
  Sum1 : Sum  Inputs=|++
  Sum2 : Sum  Inputs=|++
  m' : Outport
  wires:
  Gain/1 -> Product3/2
  Vdc/1 -> Product3/1, Sum1/1
  Product3/1 -> Sum/2
  Product2/1 -> Gain/1
  sign/1 -> Product2/2
  Sum2/1 -> Product2/1
  Product1/1 -> Sum2/2
  Product/1 -> Sum2/1
  Constant2/1 -> Product/2
  Sum1/1 -> Product/1
  Constant1/1 -> Product1/2, Sum1/2
  Sum/1 -> m'/1
  m/1 -> Sum/1, Product1/1

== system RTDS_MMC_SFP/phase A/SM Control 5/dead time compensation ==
  sign : Inport
  Vdc : Inport  Port=2
  m : Inport  Port=3
  Constant1 : Constant  Value=Vf  OutDataTypeStr=single
  Constant2 : Constant  Value=DT/Tsw  OutDataTypeStr=single
  Gain : Gain  Gain=0.5
  Product : Product
  Product1 : Product
  Product2 : Product
  Product3 : Product  Inputs=/*
  Sum : Sum  Inputs=|++
  Sum1 : Sum  Inputs=|++
  Sum2 : Sum  Inputs=|++
  m' : Outport
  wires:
  m/1 -> Product1/1, Sum/1
  Sum/1 -> m'/1
  Constant1/1 -> Sum1/2, Product1/2
  Sum1/1 -> Product/1
  Constant2/1 -> Product/2
  Product/1 -> Sum2/1
  Product1/1 -> Sum2/2
  Sum2/1 -> Product2/1
  sign/1 -> Product2/2
  Product2/1 -> Gain/1
  Product3/1 -> Sum/2
  Vdc/1 -> Sum1/1, Product3/1
  Gain/1 -> Product3/2

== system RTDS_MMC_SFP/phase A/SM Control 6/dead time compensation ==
  sign : Inport
  Vdc : Inport  Port=2
  m : Inport  Port=3
  Constant1 : Constant  Value=Vf  OutDataTypeStr=single
  Constant2 : Constant  Value=DT/Tsw  OutDataTypeStr=single
  Gain : Gain  Gain=0.5
  Product : Product
  Product1 : Product
  Product2 : Product
  Product3 : Product  Inputs=/*
  Sum : Sum  Inputs=|++
  Sum1 : Sum  Inputs=|++
  Sum2 : Sum  Inputs=|++
  m' : Outport
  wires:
  Gain/1 -> Product3/2
  Vdc/1 -> Product3/1, Sum1/1
  Product3/1 -> Sum/2
  Product2/1 -> Gain/1
  sign/1 -> Product2/2
  Sum2/1 -> Product2/1
  Product1/1 -> Sum2/2
  Product/1 -> Sum2/1
  Constant2/1 -> Product/2
  Sum1/1 -> Product/1
  Constant1/1 -> Product1/2, Sum1/2
  Sum/1 -> m'/1
  m/1 -> Sum/1, Product1/1

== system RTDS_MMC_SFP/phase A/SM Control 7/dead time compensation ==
  sign : Inport
  Vdc : Inport  Port=2
  m : Inport  Port=3
  Constant1 : Constant  Value=Vf  OutDataTypeStr=single
  Constant2 : Constant  Value=DT/Tsw  OutDataTypeStr=single
  Gain : Gain  Gain=0.5
  Product : Product
  Product1 : Product
  Product2 : Product
  Product3 : Product  Inputs=/*
  Sum : Sum  Inputs=|++
  Sum1 : Sum  Inputs=|++
  Sum2 : Sum  Inputs=|++
  m' : Outport
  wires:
  m/1 -> Product1/1, Sum/1
  Sum/1 -> m'/1
  Constant1/1 -> Sum1/2, Product1/2
  Sum1/1 -> Product/1
  Constant2/1 -> Product/2
  Product/1 -> Sum2/1
  Product1/1 -> Sum2/2
  Sum2/1 -> Product2/1
  sign/1 -> Product2/2
  Product2/1 -> Gain/1
  Product3/1 -> Sum/2
  Vdc/1 -> Sum1/1, Product3/1
  Gain/1 -> Product3/2

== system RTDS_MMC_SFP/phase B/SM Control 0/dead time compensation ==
  sign : Inport
  Vdc : Inport  Port=2
  m : Inport  Port=3
  Constant1 : Constant  Value=Vf  OutDataTypeStr=single
  Constant2 : Constant  Value=DT/Tsw  OutDataTypeStr=single
  Gain : Gain  Gain=0.5
  Product : Product
  Product1 : Product
  Product2 : Product
  Product3 : Product  Inputs=/*
  Sum : Sum  Inputs=|++
  Sum1 : Sum  Inputs=|++
  Sum2 : Sum  Inputs=|++
  m' : Outport
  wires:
  m/1 -> Product1/1, Sum/1
  Sum/1 -> m'/1
  Constant1/1 -> Sum1/2, Product1/2
  Sum1/1 -> Product/1
  Constant2/1 -> Product/2
  Product/1 -> Sum2/1
  Product1/1 -> Sum2/2
  Sum2/1 -> Product2/1
  sign/1 -> Product2/2
  Product2/1 -> Gain/1
  Product3/1 -> Sum/2
  Vdc/1 -> Sum1/1, Product3/1
  Gain/1 -> Product3/2

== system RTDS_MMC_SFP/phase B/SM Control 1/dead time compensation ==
  sign : Inport
  Vdc : Inport  Port=2
  m : Inport  Port=3
  Constant1 : Constant  Value=Vf  OutDataTypeStr=single
  Constant2 : Constant  Value=DT/Tsw  OutDataTypeStr=single
  Gain : Gain  Gain=0.5
  Product : Product
  Product1 : Product
  Product2 : Product
  Product3 : Product  Inputs=/*
  Sum : Sum  Inputs=|++
  Sum1 : Sum  Inputs=|++
  Sum2 : Sum  Inputs=|++
  m' : Outport
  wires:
  Gain/1 -> Product3/2
  Vdc/1 -> Product3/1, Sum1/1
  Product3/1 -> Sum/2
  Product2/1 -> Gain/1
  sign/1 -> Product2/2
  Sum2/1 -> Product2/1
  Product1/1 -> Sum2/2
  Product/1 -> Sum2/1
  Constant2/1 -> Product/2
  Sum1/1 -> Product/1
  Constant1/1 -> Product1/2, Sum1/2
  Sum/1 -> m'/1
  m/1 -> Sum/1, Product1/1

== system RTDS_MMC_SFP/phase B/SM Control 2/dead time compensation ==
  sign : Inport
  Vdc : Inport  Port=2
  m : Inport  Port=3
  Constant1 : Constant  Value=Vf  OutDataTypeStr=single
  Constant2 : Constant  Value=DT/Tsw  OutDataTypeStr=single
  Gain : Gain  Gain=0.5
  Product : Product
  Product1 : Product
  Product2 : Product
  Product3 : Product  Inputs=/*
  Sum : Sum  Inputs=|++
  Sum1 : Sum  Inputs=|++
  Sum2 : Sum  Inputs=|++
  m' : Outport
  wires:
  m/1 -> Product1/1, Sum/1
  Sum/1 -> m'/1
  Constant1/1 -> Sum1/2, Product1/2
  Sum1/1 -> Product/1
  Constant2/1 -> Product/2
  Product/1 -> Sum2/1
  Product1/1 -> Sum2/2
  Sum2/1 -> Product2/1
  sign/1 -> Product2/2
  Product2/1 -> Gain/1
  Product3/1 -> Sum/2
  Vdc/1 -> Sum1/1, Product3/1
  Gain/1 -> Product3/2

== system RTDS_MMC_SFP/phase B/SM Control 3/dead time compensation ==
  sign : Inport
  Vdc : Inport  Port=2
  m : Inport  Port=3
  Constant1 : Constant  Value=Vf  OutDataTypeStr=single
  Constant2 : Constant  Value=DT/Tsw  OutDataTypeStr=single
  Gain : Gain  Gain=0.5
  Product : Product
  Product1 : Product
  Product2 : Product
  Product3 : Product  Inputs=/*
  Sum : Sum  Inputs=|++
  Sum1 : Sum  Inputs=|++
  Sum2 : Sum  Inputs=|++
  m' : Outport
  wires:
  Gain/1 -> Product3/2
  Vdc/1 -> Product3/1, Sum1/1
  Product3/1 -> Sum/2
  Product2/1 -> Gain/1
  sign/1 -> Product2/2
  Sum2/1 -> Product2/1
  Product1/1 -> Sum2/2
  Product/1 -> Sum2/1
  Constant2/1 -> Product/2
  Sum1/1 -> Product/1
  Constant1/1 -> Product1/2, Sum1/2
  Sum/1 -> m'/1
  m/1 -> Sum/1, Product1/1

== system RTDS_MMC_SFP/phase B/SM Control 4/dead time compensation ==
  sign : Inport
  Vdc : Inport  Port=2
  m : Inport  Port=3
  Constant1 : Constant  Value=Vf  OutDataTypeStr=single
  Constant2 : Constant  Value=DT/Tsw  OutDataTypeStr=single
  Gain : Gain  Gain=0.5
  Product : Product
  Product1 : Product
  Product2 : Product
  Product3 : Product  Inputs=/*
  Sum : Sum  Inputs=|++
  Sum1 : Sum  Inputs=|++
  Sum2 : Sum  Inputs=|++
  m' : Outport
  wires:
  Gain/1 -> Product3/2
  Vdc/1 -> Product3/1, Sum1/1
  Product3/1 -> Sum/2
  Product2/1 -> Gain/1
  sign/1 -> Product2/2
  Sum2/1 -> Product2/1
  Product1/1 -> Sum2/2
  Product/1 -> Sum2/1
  Constant2/1 -> Product/2
  Sum1/1 -> Product/1
  Constant1/1 -> Product1/2, Sum1/2
  Sum/1 -> m'/1
  m/1 -> Sum/1, Product1/1

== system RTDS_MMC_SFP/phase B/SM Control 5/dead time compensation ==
  sign : Inport
  Vdc : Inport  Port=2
  m : Inport  Port=3
  Constant1 : Constant  Value=Vf  OutDataTypeStr=single
  Constant2 : Constant  Value=DT/Tsw  OutDataTypeStr=single
  Gain : Gain  Gain=0.5
  Product : Product
  Product1 : Product
  Product2 : Product
  Product3 : Product  Inputs=/*
  Sum : Sum  Inputs=|++
  Sum1 : Sum  Inputs=|++
  Sum2 : Sum  Inputs=|++
  m' : Outport
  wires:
  m/1 -> Product1/1, Sum/1
  Sum/1 -> m'/1
  Constant1/1 -> Sum1/2, Product1/2
  Sum1/1 -> Product/1
  Constant2/1 -> Product/2
  Product/1 -> Sum2/1
  Product1/1 -> Sum2/2
  Sum2/1 -> Product2/1
  sign/1 -> Product2/2
  Product2/1 -> Gain/1
  Product3/1 -> Sum/2
  Vdc/1 -> Sum1/1, Product3/1
  Gain/1 -> Product3/2

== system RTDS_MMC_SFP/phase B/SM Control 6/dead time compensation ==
  sign : Inport
  Vdc : Inport  Port=2
  m : Inport  Port=3
  Constant1 : Constant  Value=Vf  OutDataTypeStr=single
  Constant2 : Constant  Value=DT/Tsw  OutDataTypeStr=single
  Gain : Gain  Gain=0.5
  Product : Product
  Product1 : Product
  Product2 : Product
  Product3 : Product  Inputs=/*
  Sum : Sum  Inputs=|++
  Sum1 : Sum  Inputs=|++
  Sum2 : Sum  Inputs=|++
  m' : Outport
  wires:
  Gain/1 -> Product3/2
  Vdc/1 -> Product3/1, Sum1/1
  Product3/1 -> Sum/2
  Product2/1 -> Gain/1
  sign/1 -> Product2/2
  Sum2/1 -> Product2/1
  Product1/1 -> Sum2/2
  Product/1 -> Sum2/1
  Constant2/1 -> Product/2
  Sum1/1 -> Product/1
  Constant1/1 -> Product1/2, Sum1/2
  Sum/1 -> m'/1
  m/1 -> Sum/1, Product1/1

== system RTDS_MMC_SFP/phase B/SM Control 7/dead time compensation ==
  sign : Inport
  Vdc : Inport  Port=2
  m : Inport  Port=3
  Constant1 : Constant  Value=Vf  OutDataTypeStr=single
  Constant2 : Constant  Value=DT/Tsw  OutDataTypeStr=single
  Gain : Gain  Gain=0.5
  Product : Product
  Product1 : Product
  Product2 : Product
  Product3 : Product  Inputs=/*
  Sum : Sum  Inputs=|++
  Sum1 : Sum  Inputs=|++
  Sum2 : Sum  Inputs=|++
  m' : Outport
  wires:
  m/1 -> Product1/1, Sum/1
  Sum/1 -> m'/1
  Constant1/1 -> Sum1/2, Product1/2
  Sum1/1 -> Product/1
  Constant2/1 -> Product/2
  Product/1 -> Sum2/1
  Product1/1 -> Sum2/2
  Sum2/1 -> Product2/1
  sign/1 -> Product2/2
  Product2/1 -> Gain/1
  Product3/1 -> Sum/2
  Vdc/1 -> Sum1/1, Product3/1
  Gain/1 -> Product3/2

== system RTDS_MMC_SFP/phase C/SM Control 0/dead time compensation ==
  sign : Inport
  Vdc : Inport  Port=2
  m : Inport  Port=3
  Constant1 : Constant  Value=Vf  OutDataTypeStr=single
  Constant2 : Constant  Value=DT/Tsw  OutDataTypeStr=single
  Gain : Gain  Gain=0.5
  Product : Product
  Product1 : Product
  Product2 : Product
  Product3 : Product  Inputs=/*
  Sum : Sum  Inputs=|++
  Sum1 : Sum  Inputs=|++
  Sum2 : Sum  Inputs=|++
  m' : Outport
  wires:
  m/1 -> Product1/1, Sum/1
  Sum/1 -> m'/1
  Constant1/1 -> Sum1/2, Product1/2
  Sum1/1 -> Product/1
  Constant2/1 -> Product/2
  Product/1 -> Sum2/1
  Product1/1 -> Sum2/2
  Sum2/1 -> Product2/1
  sign/1 -> Product2/2
  Product2/1 -> Gain/1
  Product3/1 -> Sum/2
  Vdc/1 -> Sum1/1, Product3/1
  Gain/1 -> Product3/2

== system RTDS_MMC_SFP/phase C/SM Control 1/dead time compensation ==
  sign : Inport
  Vdc : Inport  Port=2
  m : Inport  Port=3
  Constant1 : Constant  Value=Vf  OutDataTypeStr=single
  Constant2 : Constant  Value=DT/Tsw  OutDataTypeStr=single
  Gain : Gain  Gain=0.5
  Product : Product
  Product1 : Product
  Product2 : Product
  Product3 : Product  Inputs=/*
  Sum : Sum  Inputs=|++
  Sum1 : Sum  Inputs=|++
  Sum2 : Sum  Inputs=|++
  m' : Outport
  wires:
  Gain/1 -> Product3/2
  Vdc/1 -> Product3/1, Sum1/1
  Product3/1 -> Sum/2
  Product2/1 -> Gain/1
  sign/1 -> Product2/2
  Sum2/1 -> Product2/1
  Product1/1 -> Sum2/2
  Product/1 -> Sum2/1
  Constant2/1 -> Product/2
  Sum1/1 -> Product/1
  Constant1/1 -> Product1/2, Sum1/2
  Sum/1 -> m'/1
  m/1 -> Sum/1, Product1/1

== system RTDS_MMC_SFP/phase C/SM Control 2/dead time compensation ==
  sign : Inport
  Vdc : Inport  Port=2
  m : Inport  Port=3
  Constant1 : Constant  Value=Vf  OutDataTypeStr=single
  Constant2 : Constant  Value=DT/Tsw  OutDataTypeStr=single
  Gain : Gain  Gain=0.5
  Product : Product
  Product1 : Product
  Product2 : Product
  Product3 : Product  Inputs=/*
  Sum : Sum  Inputs=|++
  Sum1 : Sum  Inputs=|++
  Sum2 : Sum  Inputs=|++
  m' : Outport
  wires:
  m/1 -> Product1/1, Sum/1
  Sum/1 -> m'/1
  Constant1/1 -> Sum1/2, Product1/2
  Sum1/1 -> Product/1
  Constant2/1 -> Product/2
  Product/1 -> Sum2/1
  Product1/1 -> Sum2/2
  Sum2/1 -> Product2/1
  sign/1 -> Product2/2
  Product2/1 -> Gain/1
  Product3/1 -> Sum/2
  Vdc/1 -> Sum1/1, Product3/1
  Gain/1 -> Product3/2

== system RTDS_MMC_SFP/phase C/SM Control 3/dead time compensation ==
  sign : Inport
  Vdc : Inport  Port=2
  m : Inport  Port=3
  Constant1 : Constant  Value=Vf  OutDataTypeStr=single
  Constant2 : Constant  Value=DT/Tsw  OutDataTypeStr=single
  Gain : Gain  Gain=0.5
  Product : Product
  Product1 : Product
  Product2 : Product
  Product3 : Product  Inputs=/*
  Sum : Sum  Inputs=|++
  Sum1 : Sum  Inputs=|++
  Sum2 : Sum  Inputs=|++
  m' : Outport
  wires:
  Gain/1 -> Product3/2
  Vdc/1 -> Product3/1, Sum1/1
  Product3/1 -> Sum/2
  Product2/1 -> Gain/1
  sign/1 -> Product2/2
  Sum2/1 -> Product2/1
  Product1/1 -> Sum2/2
  Product/1 -> Sum2/1
  Constant2/1 -> Product/2
  Sum1/1 -> Product/1
  Constant1/1 -> Product1/2, Sum1/2
  Sum/1 -> m'/1
  m/1 -> Sum/1, Product1/1

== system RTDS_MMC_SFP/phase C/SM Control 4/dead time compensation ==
  sign : Inport
  Vdc : Inport  Port=2
  m : Inport  Port=3
  Constant1 : Constant  Value=Vf  OutDataTypeStr=single
  Constant2 : Constant  Value=DT/Tsw  OutDataTypeStr=single
  Gain : Gain  Gain=0.5
  Product : Product
  Product1 : Product
  Product2 : Product
  Product3 : Product  Inputs=/*
  Sum : Sum  Inputs=|++
  Sum1 : Sum  Inputs=|++
  Sum2 : Sum  Inputs=|++
  m' : Outport
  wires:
  Gain/1 -> Product3/2
  Vdc/1 -> Product3/1, Sum1/1
  Product3/1 -> Sum/2
  Product2/1 -> Gain/1
  sign/1 -> Product2/2
  Sum2/1 -> Product2/1
  Product1/1 -> Sum2/2
  Product/1 -> Sum2/1
  Constant2/1 -> Product/2
  Sum1/1 -> Product/1
  Constant1/1 -> Product1/2, Sum1/2
  Sum/1 -> m'/1
  m/1 -> Sum/1, Product1/1

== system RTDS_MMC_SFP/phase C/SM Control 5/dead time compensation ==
  sign : Inport
  Vdc : Inport  Port=2
  m : Inport  Port=3
  Constant1 : Constant  Value=Vf  OutDataTypeStr=single
  Constant2 : Constant  Value=DT/Tsw  OutDataTypeStr=single
  Gain : Gain  Gain=0.5
  Product : Product
  Product1 : Product
  Product2 : Product
  Product3 : Product  Inputs=/*
  Sum : Sum  Inputs=|++
  Sum1 : Sum  Inputs=|++
  Sum2 : Sum  Inputs=|++
  m' : Outport
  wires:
  m/1 -> Product1/1, Sum/1
  Sum/1 -> m'/1
  Constant1/1 -> Sum1/2, Product1/2
  Sum1/1 -> Product/1
  Constant2/1 -> Product/2
  Product/1 -> Sum2/1
  Product1/1 -> Sum2/2
  Sum2/1 -> Product2/1
  sign/1 -> Product2/2
  Product2/1 -> Gain/1
  Product3/1 -> Sum/2
  Vdc/1 -> Sum1/1, Product3/1
  Gain/1 -> Product3/2
